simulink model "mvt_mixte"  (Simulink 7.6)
settings: Solver=ode15s  StartTime=0.0  StopTime=1.5  RelTol=1e-3
InitFcn:
  | clc
  | clear all
  | close all
StopFcn:
  | close all, clc
  | load mvt_rotation.mat
  | plotyy(x(1,:),x(2,:),x(1,:),x(3,:))
  | title('Position et vitesse de rotation')
  | xlabel('temps')
  | grid
  | 
  | figure
  | 
  | load mvt_translation.mat
  | plotyy(y(1,:),y(2,:),y(1,:),y(3,:))
  | title('Position et vitesse de translation')
  | xlabel('temps')
  | grid
  | 
  | delete *.mat
libraries: fl_lib x11, nesl_utility x6

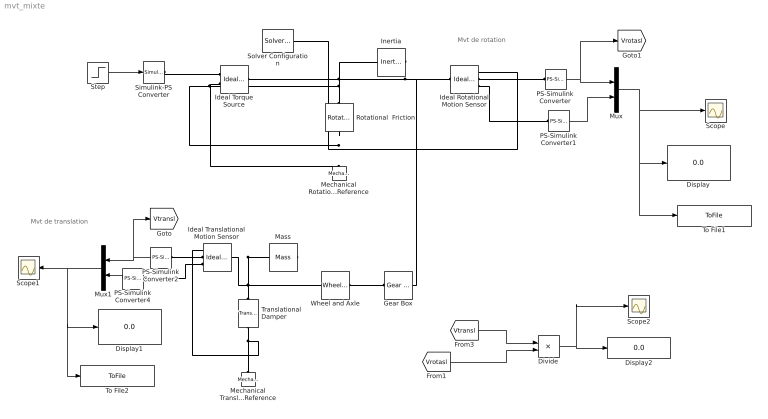
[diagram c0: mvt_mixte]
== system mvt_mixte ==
  note: Mvt de rotation
  note: Mvt de translation
  Display : Display
  Display1 : Display
  Display2 : Display
  Divide : Product  Inputs=*/
  Gear Box : fl_lib/Mechanical/Mechanisms/Gear Box  DialogController=NetworkEngine.DynNeDlgSource  SystemSampleTime=-1  ratio=5  t_in_Log=off  t_out_Log=off  LocalVarNames=|t_in|t_out  LocalVarDescs=|t_in|t_out  LocalVarLogging=[0 0]
  Ideal Rotational Motion Sensor : fl_lib/Mechanical/Mechanical Sensors/Ideal Rotational Motion Sensor  DialogController=NetworkEngine.DynNeDlgSource  SystemSampleTime=-1  offset=0 rad  w_Log=off  t_Log=off  phi_Log=off  LocalVarNames=|w|t|phi  LocalVarDescs=|w|t|phi  LocalVarLogging=[0 0 0]
  Ideal Torque Source : fl_lib/Mechanical/Mechanical Sources/Ideal Torque Source  DialogController=NetworkEngine.DynNeDlgSource  SystemSampleTime=-1  w_Log=off  t_Log=off  LocalVarNames=|w|t  LocalVarDescs=|w|t  LocalVarLogging=[0 0]
  Ideal Translational Motion Sensor : fl_lib/Mechanical/Mechanical Sensors/Ideal Translational Motion Sensor  DialogController=NetworkEngine.DynNeDlgSource  SystemSampleTime=-1  offset=0 m  v_Log=off  f_Log=off  x_Log=off  LocalVarNames=|v|f|x  LocalVarDescs=|v|f|x  LocalVarLogging=[0 0 0]
  Inertia : fl_lib/Mechanical/Rotational Elements/Inertia  DialogController=NetworkEngine.DynNeDlgSource  SystemSampleTime=-1  inertia=0.01 kg*m^2  initial_velocity=0 rad/s  t_Log=off  LocalVarNames=|t  LocalVarDescs=|t  LocalVarLogging=0
  Mass : fl_lib/Mechanical/Translational Elements/Mass  DialogController=NetworkEngine.DynNeDlgSource  SystemSampleTime=-1  mass=1 kg  initial_velocity=0 m/s  f_Log=off  LocalVarNames=|f  LocalVarDescs=|f  LocalVarLogging=0
  Mechanical Rotational Reference : fl_lib/Mechanical/Rotational Elements/Mechanical Rotational Reference  DialogController=NetworkEngine.DynNeDlgSource  SystemSampleTime=-1  t_Log=off  LocalVarNames=|t  LocalVarDescs=|t  LocalVarLogging=0
  Mechanical Translational Reference : fl_lib/Mechanical/Translational Elements/Mechanical Translational Reference  DialogController=NetworkEngine.DynNeDlgSource  SystemSampleTime=-1  f_Log=off  LocalVarNames=|f  LocalVarDescs=|f  LocalVarLogging=0
  Mux : Mux  Inputs=2
  Mux1 : Mux  Inputs=2
  PS-Simulink Converter{,1..2,4} (4 alike) : nesl_utility/PS-Simulink Converter  DialogController=NetworkEngine.DynNeUtilDlgSource  SystemSampleTime=-1  PhysicalDomain=network_engine_domain  LeftPortType=input  RightPortType=output  SubClassName=ps_output  Unit=1  AffineConversion=off
  Rotational  Friction : fl_lib/Mechanical/Rotational Elements/Rotational Friction  DialogController=NetworkEngine.DynNeDlgSource  SystemSampleTime=-1  brkwy_trq=0.001 N*m  Col_trq=0.00001 N*m  visc_coef=0.1 N*m/(rad/s)  trans_coef=10 s/rad  vel_thr=1e-4 rad/s  t_Log=off  w_Log=off  LocalVarNames=|t|w  LocalVarDescs=|t|w  LocalVarLogging=[0 0]
  Scope : Scope
  Scope1 : Scope
  Scope2 : Scope
  Simulink-PS Converter : nesl_utility/Simulink-PS Converter  DialogController=NetworkEngine.DynNeUtilDlgSource  SystemSampleTime=-1  PhysicalDomain=network_engine_domain  LeftPortType=input  RightPortType=output  SubClassName=ps_input  Unit=1  AffineConversion=off  InputFilterTimeConstant=.001  UdotUserProvided=0
  Solver Configuration : nesl_utility/Solver Configuration  DialogController=NetworkEngine.DynNeUtilDlgSource  SystemSampleTime=-1  PhysicalDomain=network_engine_domain  LeftPortType=input  RightPortType=generic  SubClassName=solver  Accelerate=off  Profile=off  ResidualTolerance=1e-9  MaxNonlinIter=3  MaxModeIter=2  DoFixedCost=off  UseLocalSampling=off  DoDC=off  LinearAlgebra=Sparse  LocalSolverSampleTime=.001  LocalSolverChoice=NE_BACKWARD_EULER_ADVANCER  UseLocalSolver=off
  Step : Step  Time=0.2  After=1000  SampleTime=0
  To File1 : ToFile  Filename=mvt_rotation  MatrixName=x
  To File2 : ToFile  Filename=mvt_translation  MatrixName=y
  Translational  Damper : fl_lib/Mechanical/Translational Elements/Translational Damper  DialogController=NetworkEngine.DynNeDlgSource  SystemSampleTime=-1  D=100 N/(m/s)  f_Log=off  v_Log=off  LocalVarNames=|f|v  LocalVarDescs=|f|v  LocalVarLogging=[0 0]
  Wheel and Axle : fl_lib/Mechanical/Mechanisms/Wheel and Axle  DialogController=NetworkEngine.DynNeDlgSource  SystemSampleTime=-1  R=0.05 m  or=1  torque_A_Log=off  force_P_Log=off  ang_velocity_Log=off  velocity_Log=off  LocalVarNames=|torque_A|force_P|ang_velocity|velocity  LocalVarDescs=|Axle torque (N*m)|Periphery force (N)|Axle angular velocity (rad/s)|Periphery velocity (m/s)  LocalVarLogging=[0 0 0 0]
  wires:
  Step/1 -> Simulink-PS Converter/1
  PS-Simulink Converter/1 -> Mux/1, [Vrotasl]
  PS-Simulink Converter1/1 -> Mux/2
  Mux/1 -> Display/1, To File1/1, Scope/1
  PS-Simulink Converter2/1 -> Mux1/1, [Vtransl]
  PS-Simulink Converter4/1 -> Mux1/2
  Mux1/1 -> Scope1/1, Display1/1, To File2/1
  [Vtransl] -> Divide/1
  [Vrotasl] -> Divide/2
  Divide/1 -> Display2/1, Scope2/1
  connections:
  Ideal Torque Source/RConn2 -- Rotational  Friction/RConn1 -- Mechanical Rotational Reference/LConn1 -- Ideal Rotational Motion Sensor/RConn1
  Ideal Torque Source/LConn1 -- Inertia/LConn1 -- Ideal Rotational Motion Sensor/LConn1 -- Gear Box/RConn1 -- Rotational  Friction/LConn1 -- Solver Configuration/RConn1
  Simulink-PS Converter/RConn1 -- Ideal Torque Source/RConn1
  Ideal Rotational Motion Sensor/RConn2 -- PS-Simulink Converter/LConn1
  Ideal Rotational Motion Sensor/RConn3 -- PS-Simulink Converter1/LConn1
  Translational  Damper/RConn1 -- Mechanical Translational Reference/LConn1 -- Ideal Translational Motion Sensor/RConn1
  Ideal Translational Motion Sensor/LConn1 -- Mass/LConn1 -- Translational  Damper/LConn1 -- Wheel and Axle/RConn1
  PS-Simulink Converter2/LConn1 -- Ideal Translational Motion Sensor/RConn2
  Ideal Translational Motion Sensor/RConn3 -- PS-Simulink Converter4/LConn1
  Wheel and Axle/LConn1 -- Gear Box/LConn1
